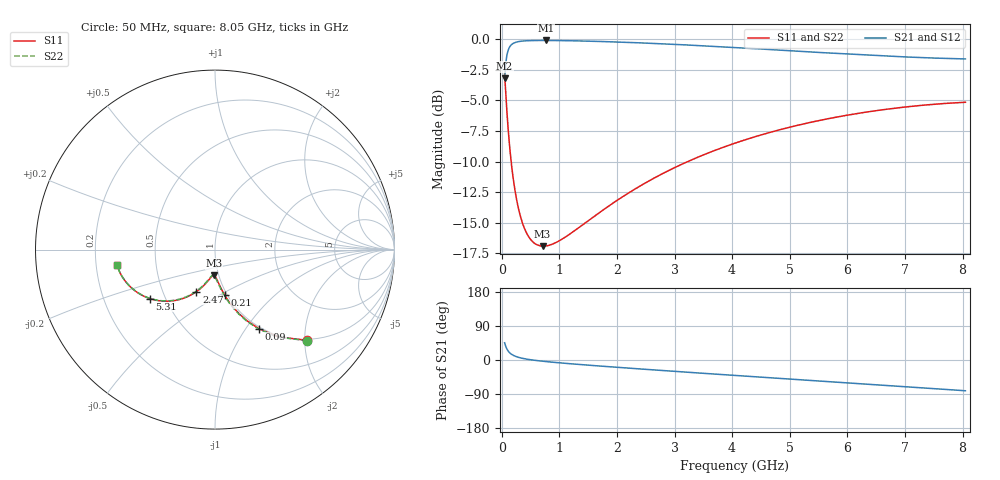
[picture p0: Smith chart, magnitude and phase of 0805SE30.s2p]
! AVX Thin Film Operation		Date: August 2001
! Description: Accu-P® Series, Thin Film, SMD, RF Capacitor
! Part Number: 08053J300FBT
! 50 MHz  -  8.05 GHz
! Serial Measurements
# mhz S db R 50
!	S11		S21		S12		S22
!	dB	Phase	dB	Phase	dB	Phase	dB	Phase
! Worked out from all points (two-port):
!   401 points, 50 MHz to 8.05 GHz, reference 50 ohm
!   highest |S21| = -0.09 dB at 770 MHz (marker M1); lowest = -3.2 dB at 50 MHz (marker M2)
!   |S21| within 3 dB of the highest: 51.67 MHz to end of sweep
!   lowest |S11| = -16.9 dB at 710 MHz (marker M3), VSWR 1.33, Z = 47.4 - j13.8 ohm
!   |S11| at or under -10 dB: 164 MHz to 3.23 GHz (3.066 GHz wide, 181 % of centre)
!   |S22| runs from -16.9 to -2.8 dB; largest |S21 - S12| = 0
!   S11 on the Smith chart (normalised r, x): 50 MHz: 0.97, -2.06; 90 MHz: 0.97, -1.16; 210 MHz: 0.97, -0.53; 2.47 GHz: 0.73, -0.37; 5.31 GHz: 0.41, -0.28; 8.05 GHz: 0.29, -0.07
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50  -2.83 -44.5  -3.20 45.4  -3.20 45.4  -2.83 -44.7
90  -5.92 -60.9  -1.29 28.9  -1.29 28.9  -5.92 -61.2
110  -7.24 -65.8  -0.91 24.0  -0.91 24.0  -7.24 -66.1
130  -8.38 -69.4  -0.69 20.3  -0.69 20.3  -8.38 -69.9
170  -10.27 -74.6  -0.43 15.1  -0.43 15.1  -10.27 -75.1
210  -11.73 -78.0  -0.30 11.6  -0.30 11.6  -11.73 -78.6
250  -12.90 -80.5  -0.23 9.1  -0.23 9.1  -12.90 -81.2
310  -14.22 -83.3  -0.17 6.2  -0.17 6.2  -14.22 -84.1
410  -15.64 -86.5  -0.12 2.9  -0.12 2.9  -15.64 -87.5
550  -16.62 -89.7  -0.10 -0.4  -0.10 -0.4  -16.62 -90.8
710  -16.92 -92.5  -0.09 -3.2  -0.09 -3.2  -16.92 -93.7
770  -16.91 -93.5  -0.09 -4.2  -0.09 -4.2  -16.91 -94.6
1010  -16.45 -96.9  -0.10 -7.6  -0.10 -7.6  -16.45 -98.0
1390  -15.23 -101.7  -0.14 -12.3  -0.14 -12.3  -15.23 -102.7
2470  -11.81 -113.9  -0.30 -24.3  -0.30 -24.3  -11.81 -114.5
2730  -11.14 -116.7  -0.35 -27.1  -0.35 -27.1  -11.14 -117.3
3370  -9.71 -123.4  -0.50 -33.8  -0.50 -33.8  -9.71 -123.9
4050  -8.49 -130.4  -0.67 -40.7  -0.67 -40.7  -8.49 -130.8
5310  -6.85 -143.2  -1.02 -53.4  -1.02 -53.4  -6.85 -143.4
5390  -6.76 -144.0  -1.04 -54.2  -1.04 -54.2  -6.76 -144.2
6730  -5.69 -157.4  -1.38 -67.6  -1.38 -67.6  -5.69 -157.6
8050  -5.15 -170.9  -1.60 -81.2  -1.60 -81.2  -5.15 -171.1
